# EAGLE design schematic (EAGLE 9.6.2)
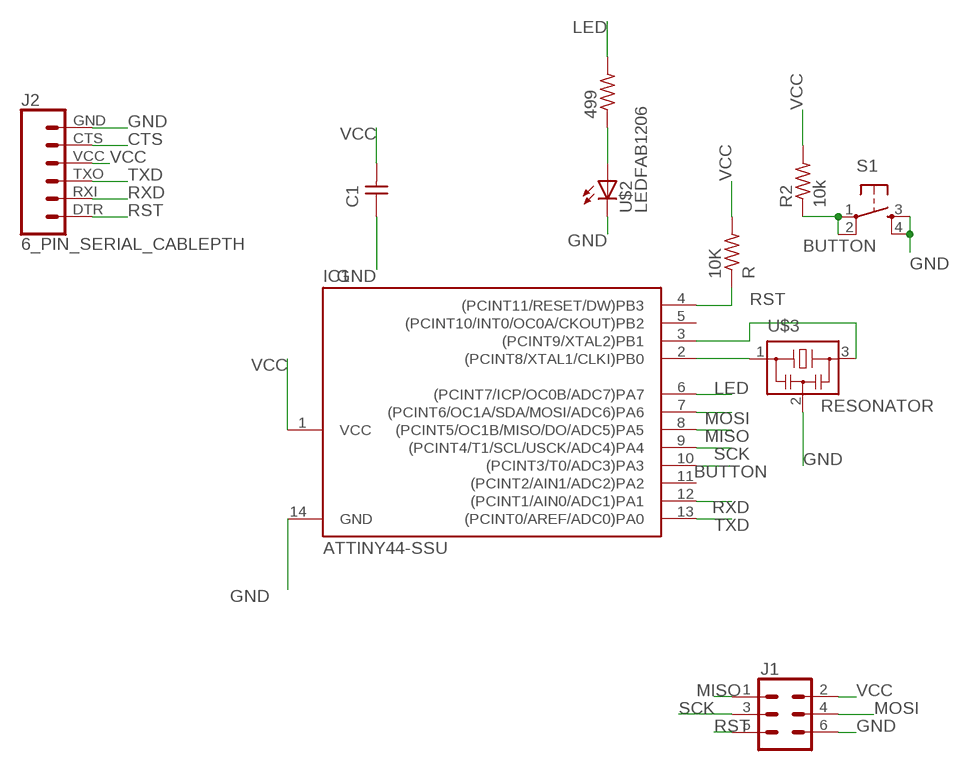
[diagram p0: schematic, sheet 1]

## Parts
10K  R  RES-US1206FAB  [R1206FAB]
499  RES-US1206FAB  [R1206FAB]
C1  CAP-UNPOLARIZEDFAB  [C1206FAB]
IC1  ATTINY44-SSU  [SOIC14]
J1  CONN_03X22X3_SILK_MALE_PTH  [2X3]
J2  6_PIN_SERIAL_CABLEPTH  [FTDI_BASIC]
R2  10k  RES-US1206FAB  [R1206FAB]
S1  6MM_SWITCH6MM_SWITCH  [6MM_SWITCH]
U$2  LEDFAB1206  [LED1206FAB]
U$3  RESONATOR  [EFOBM]

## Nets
BUTTON: IC1.10((PCINT3/T0/ADC3)PA3) R2.1 S1.1(P) S1.2(P1)
CTS: J2.CTS
GND: C1.1 IC1.14(GND) J1.6 J2.GND S1.3(S) S1.4(S1) U$2.2(C) U$3.2
LED: 499.2 IC1.6((PCINT7/ICP/OC0B/ADC7)PA7)
MISO: IC1.8((PCINT5/OC1B/MISO/DO/ADC5)PA5) J1.1
MOSI: IC1.7((PCINT6/OC1A/SDA/MOSI/ADC6)PA6) J1.4
N$4: IC1.2((PCINT8/XTAL1/CLKI)PB0) U$3.1
N$5: IC1.3((PCINT9/XTAL2)PB1) U$3.3
N$6: 499.1 U$2.1(A)
RST: 10K.1 IC1.4((PCINT11/RESET/DW)PB3) J1.5 J2.DTR
RXD: IC1.12((PCINT1/AIN0/ADC1)PA1) J2.RXI
SCK: IC1.9((PCINT4/T1/SCL/USCK/ADC4)PA4) J1.3
TXD: IC1.13((PCINT0/AREF/ADC0)PA0) J2.TXO
VCC: 10K.2 C1.2 IC1.1(VCC) J1.2 J2.VCC R2.2
Unconnected: IC1.5((PCINT10/INT0/OC0A/CKOUT)PB2) IC1.11((PCINT2/AIN1/ADC2)PA2)

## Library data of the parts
10K 499 R2 = fab:RES-US: Resistor (US Symbol)
C1 = fab:CAP-UNPOLARIZED
IC1 = fab:ATTINY44
J1 = SparkFun-Connectors:CONN_03X2: Multi connection point. Often used as Generic Header-pin footprint for 0.1 inch spaced/style header connections You can populate with any combo of single row headers, but if you'd like an exact match, check these: Header - 2x3 (Male, 0.1") (PRT-12807) Header - 2x3 (Female, 0.1") (PRT-13010) 2x3 Pin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; PROD_ID: CONN-09701
J2 = SparkFun-Connectors:6_PIN_SERIAL_CABLE: 6-pin header connection for use with the "FTDI BASIC" pinout - CABLE SIDE. Also known as "Arduino Serial Program Header". This is used on a design to provide a 6-pin connection point for serial communication usually from a USB cable (D+/D-) to these headers (RX/TX). It also has the remaining pins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
S1 = fab:6MM_SWITCH: OMRON SWITCH
U$2 = fab:LED: LED
U$3 = fab:RESONATOR

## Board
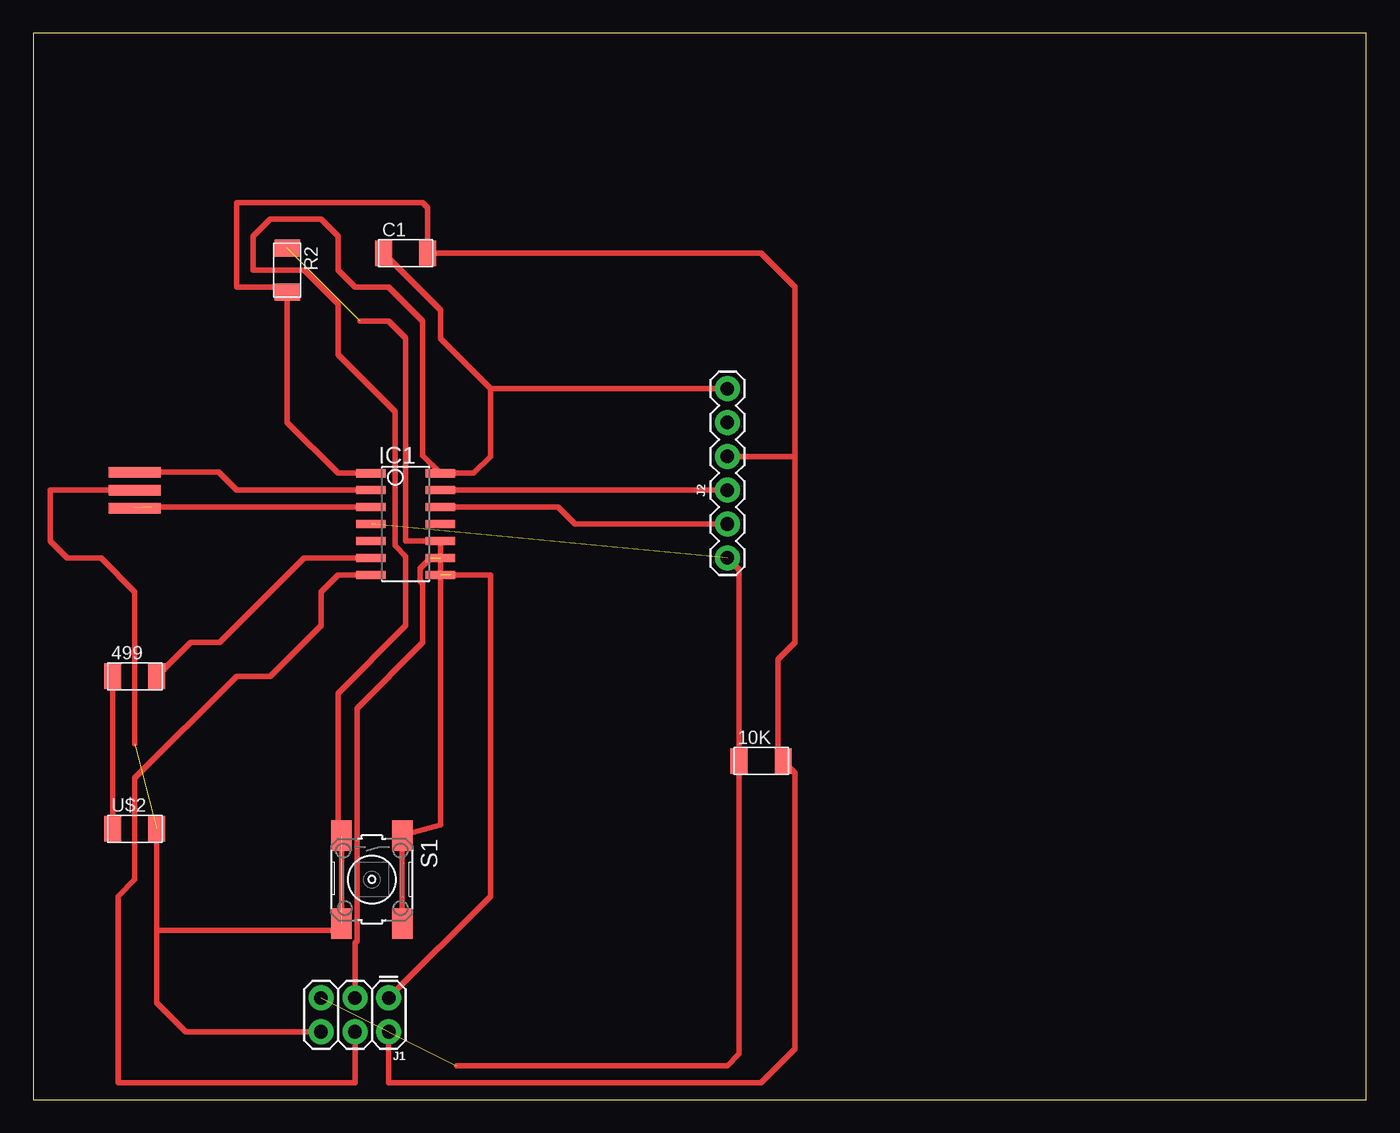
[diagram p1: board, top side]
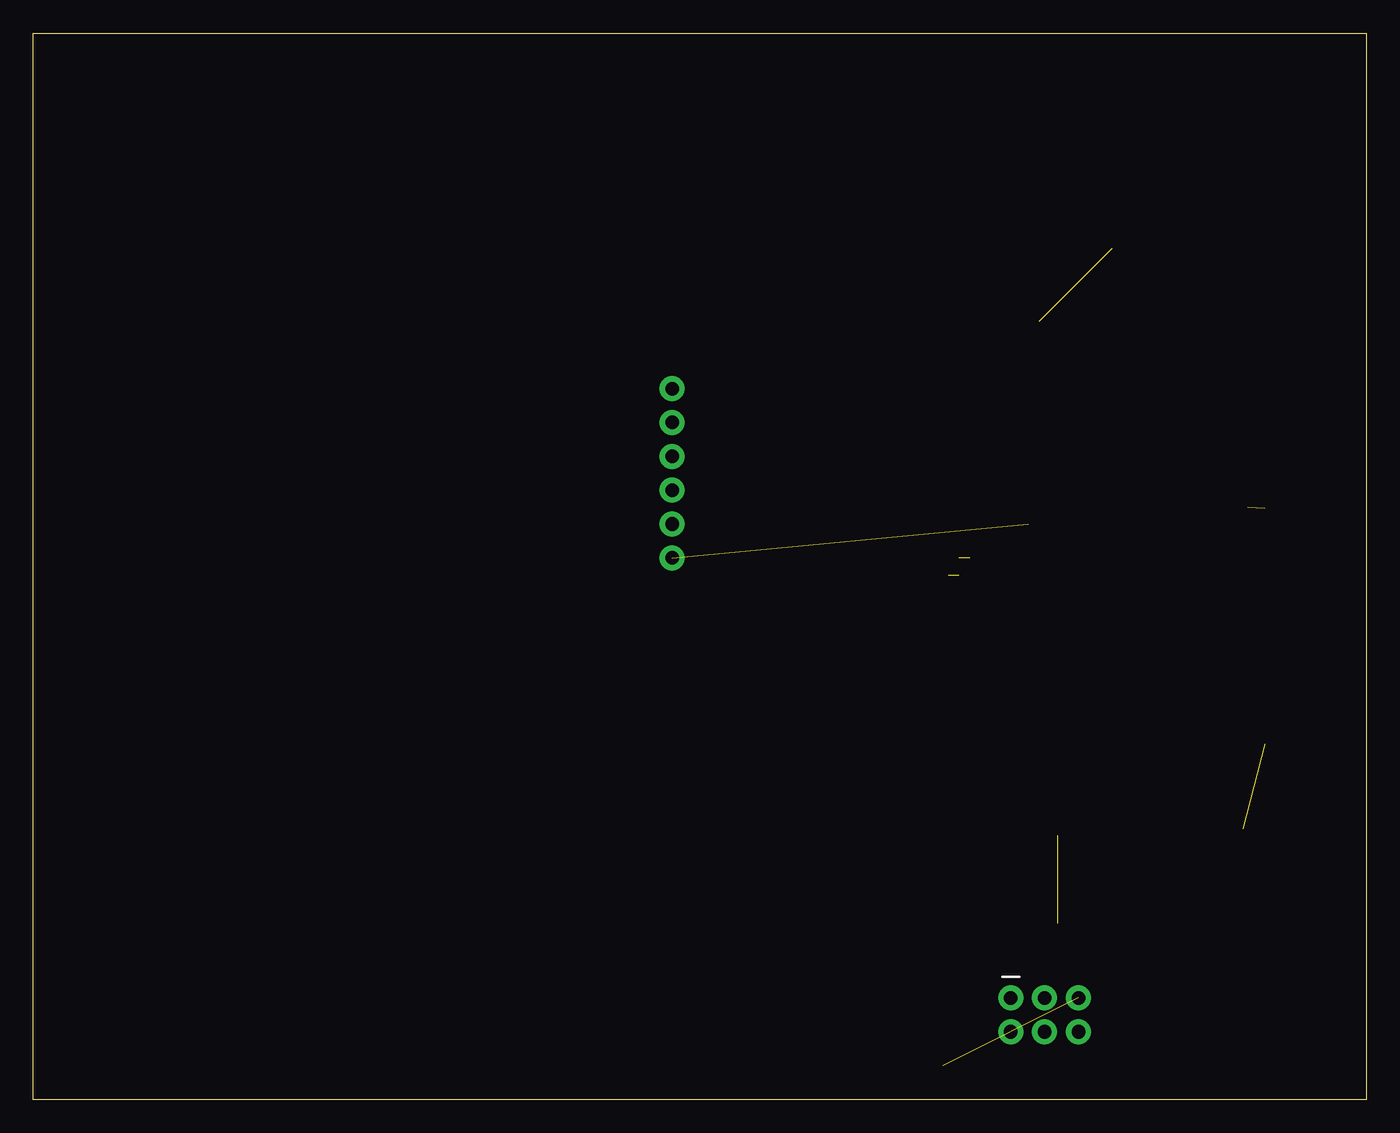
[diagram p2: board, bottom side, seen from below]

Size 100 x 80 mm. Coordinates in mm from the lower left corner, seen from the top.
Outline: 0,0 100,0 100,80 0,80 0,0
Copper layers (1*16): Top 0.035mm / dielectric 1.5mm / Bottom 0.035mm
Design rules "default *": minimum track width 6mil, minimum drill 0.35mm, track to track 16mil, track to pad 8mil, pad to pad 8mil, via to via 8mil, smd to smd 8mil, copper to edge 40mil, drill to drill 6mil, minimum pad ring 10mil, minimum via ring 8mil, stop-mask expansion 4mil, vias tented up to drill 0mil, thermal gap 10mil

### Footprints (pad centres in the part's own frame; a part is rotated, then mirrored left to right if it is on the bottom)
R1206FAB = smd 1.27 x 1.905: 1 -1.651,0; 2 1.651,0
C1206FAB = smd 1.27 x 1.905: 1 -1.651,0; 2 1.651,0
SOIC14 = smd 0.61 x 2.21: 1 -3.81,-2.603; 2 -2.54,-2.603; 3 -1.27,-2.603; 4 0,-2.603; 5 1.27,-2.603; 6 2.54,-2.603; 7 3.81,-2.603; 8 3.81,2.603; 9 2.54,2.603; 10 1.27,2.603; 11 0,2.603; 12 -1.27,2.603; 13 -2.54,2.603; 14 -3.81,2.603
2X3 = drill 1.016 pad 1.88: 1 0,0; 2 0,2.54; 3 2.54,0; 4 2.54,2.54; 5 5.08,0; 6 5.08,2.54
FTDI_BASIC = drill 1.016 pad 1.88: CTS 10.16,0; DTR 0,0; GND 12.7,0; RXI 2.54,0; TXO 5.08,0; VCC 7.62,0
6MM_SWITCH = smd 2.286 x 1.524: 1 -3.302,2.286; 2 3.302,2.286; 3 -3.302,-2.286; 4 3.302,-2.286
LED1206FAB = smd 1.27 x 1.905: 1 -1.651,0; 2 1.651,0
EFOBM = smd 0.8 x 3.9: 1 -1.35,0; 2 0,0; 3 1.35,0

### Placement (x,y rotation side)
10K  54.61,25.4 0 top
499  7.62,31.75 0 top
C1  27.94,63.5 0 top
IC1  27.94,43.18 270 top
J1  26.67,7.62 180 top
J2  52.07,40.64 90 top
R2  19.05,62.23 270 top
S1  25.4,16.51 270 top
U$2  7.62,20.32 0 top
U$3  7.62,45.72 270 top

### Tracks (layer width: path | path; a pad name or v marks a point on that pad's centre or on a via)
BUTTON  (1 unrouted)
  Top 0.406: S1.2 S1.1 30.54,20.6 IC1.10 27.94,41.91 27.94,57.15 26.67,58.42 24.51,58.42
GND  (2 unrouted)
  Top 0.406: C1.1 30.54,59.24 30.54,57.09 34.29,53.34 | 34.29,53.34 34.29,48.26 33.02,46.99 IC1.14 29.21,48.32 29.21,58.42 26.67,60.96 24.13,60.96 22.86,62.23 22.86,64.77 21.59,66.04 17.78,66.04 16.51,64.77 16.51,62.23 20.32,62.23 22.86,59.69 22.86,55.88 27.13,51.61 27.13,41.57 27.94,40.76 27.94,35.56 22.86,30.48 22.86,19.05 23.11,18.8 S1.4 22.61,12.7 9.27,12.7 | J2.GND 34.29,53.34 | J1.6 11.43,5.08 9.27,7.24 9.27,12.7 | 9.27,12.7 U$2.2 | U$3.2 1.27,45.72 1.27,41.91 2.54,40.64 5.08,40.64 7.62,38.1 7.62,26.67
LED
  Top 0.406: IC1.6 20.32,40.64 13.97,34.29 11.81,34.29 499.2
MISO  (1 unrouted)
  Top 0.406: J1.1 34.29,15.24 34.29,39.37 31.36,39.37
MOSI
  Top 0.406: J1.4 24.13,1.27 6.35,1.27 6.35,15.24 7.62,16.51 7.62,24.13 15.24,31.75 17.78,31.75 21.59,35.56 21.59,38.1 22.86,39.37 IC1.7
N$4
  Top 0.406: IC1.2 15.24,45.72 13.89,47.07 U$3.1
N$5  (1 unrouted)
  Top 0.406: IC1.3 8.89,44.45
N$6
  Top 0.406: 499.1 U$2.1
RST  (2 unrouted)
  Top 0.406: J2.DTR 52.96,39.75 10K.1 52.96,3.43 52.07,2.54 31.75,2.54
RXD
  Top 0.406: IC1.12 39.37,44.45 40.64,43.18 J2.RXI
SCK  (1 unrouted)
  Top 0.406: J1.3 24.13,11.74 24.28,11.9 24.28,29.36 29.21,34.29 29.21,38.72 29.03,38.9 29.03,39.84 29.73,40.54 29.73,40.64
TXD
  Top 0.406: IC1.13 J2.TXO
VCC
  Top 0.406: IC1.1 22.86,46.99 19.05,50.8 R2.2 18.67,60.96 15.24,60.96 15.24,67.31 29.21,67.31 29.59,66.93 C1.2 54.61,63.5 57.15,60.96 57.15,48.26 | J2.VCC 57.15,48.26 | 57.15,48.26 57.15,34.29 55.88,33.02 55.88,25.78 56.07,25.59 10K.2 57.15,24.51 57.15,3.81 54.61,1.27 26.67,1.27 J1.2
